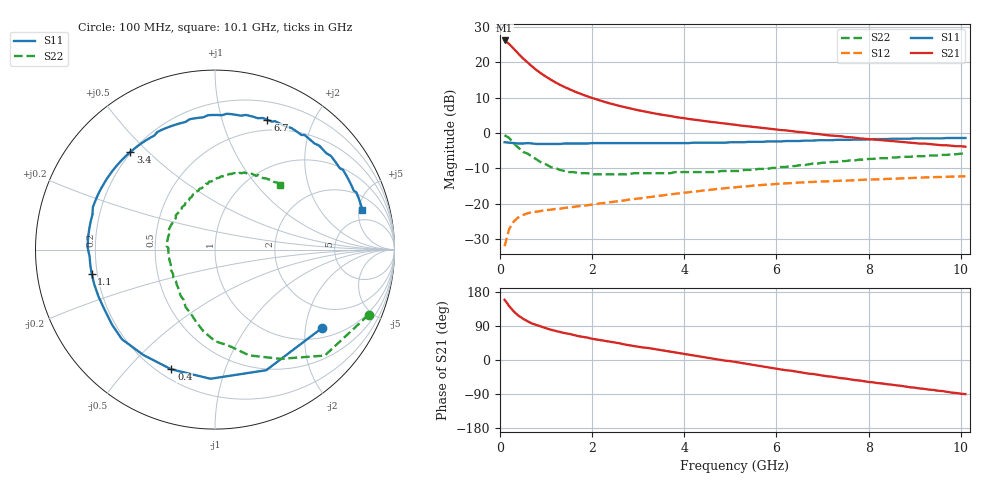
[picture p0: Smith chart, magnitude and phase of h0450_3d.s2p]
!HBFP-0450
!S and NOISE PARAMETERS at Vce=3V  Ic=10mA.  LAST UPDATED  09-04-98
# GHZ S MA R  50
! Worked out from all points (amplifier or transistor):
!   101 points, 100 MHz to 10.1 GHz, reference 50 ohm
!   highest |S21| = 26.2 dB at 100 MHz (marker M1)
!   |S21| within 3 dB of that: start of sweep to 345 MHz
!   unconditionally stable (mu >= 1): 2.623 GHz to end of sweep
!   at 1.7 GHz: K = 0.77, MSG = 16.0 dB, |S12| = -20.7 dB
!   at 5.1 GHz: K = 1.16, MAG = 6.5 dB, |S12| = -15.4 dB
!   at 10.1 GHz: K = 1.09, MAG = 2.3 dB, |S12| = -12.3 dB
!   lowest NFmin = 1.11 dB at 1.8 GHz
!   S11 on the Smith chart (normalised r, x): 100 MHz: 1.29, -2.48; 400 MHz: 0.25, -0.67; 1.1 GHz: 0.18, -0.09; 3.4 GHz: 0.20, +0.44; 6.7 GHz: 0.38, +1.41; 10.1 GHz: 3.45, +5.47
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0.1  0.74 -36.0  20.43 159.0  0.025 72.0  0.93 -23.0
0.2  0.73 -67.0  18.15 142.0  0.044 57.0  0.85 -44.0
0.3  0.72 -92.0  15.54 128.0  0.056 48.0  0.71 -59.0
0.4  0.71 -110.0  13.25 117.0  0.064 40.0  0.62 -72.0
0.5  0.71 -124.0  11.36 109.0  0.069 35.0  0.54 -82.0
0.6  0.72 -136.0  9.97 102.0  0.073 31.0  0.51 -90.0
0.7  0.71 -144.0  8.72 96.0  0.076 29.0  0.46 -98.0
0.8  0.7 -152.0  7.71 92.0  0.077 27.0  0.42 -104.0
0.9  0.7 -158.0  6.91 88.0  0.079 26.0  0.38 -111.0
1.1  0.7 -169.0  5.7 80.0  0.082 24.0  0.33 -122.0
1.4  0.71 179.0  4.48 71.0  0.087 23.0  0.29 -137.0
1.8  0.71 167.0  3.48 61.0  0.093 22.0  0.27 -153.0
2.2  0.72 156.0  2.85 52.0  0.101 21.0  0.26 -167.0
2.7  0.72 145.0  2.33 41.0  0.111 19.0  0.26 -180.0
3.4  0.72 131.0  1.87 28.0  0.128 15.0  0.27 166.0
3.5  0.72 129.0  1.82 26.0  0.13 15.0  0.27 164.0
4.3  0.73 114.0  1.52 10.0  0.15 8.0  0.28 149.0
5.1  0.74 99.0  1.31 -5.0  0.17 -1.0  0.29 133.0
6.7  0.78 68.0  1 -36.0  0.202 -21.0  0.36 100.0
6.8  0.78 66.0  0.98 -37.0  0.203 -22.0  0.37 98.0
8.5  0.83 39.0  0.77 -65.0  0.225 -43.0  0.45 72.0
10.1  0.85 15.0  0.64 -90.0  0.243 -65.0  0.51 45.0
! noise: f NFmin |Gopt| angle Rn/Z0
1.8  1.11  0.46  180  0.05
2  1.17  0.49  -176  0.05
2.5  1.33  0.53  -160  0.06
3.5  1.65  0.6  -137  0.16
4  1.82  0.63  -125  0.26
5  2.15  0.68  -103  0.57
5.5  2.32  0.71  -92  0.83
7  2.8  0.76  -63  1.93
8  3.14  0.8  -46  2.95
10  3.76  0.81  -15  5.02
